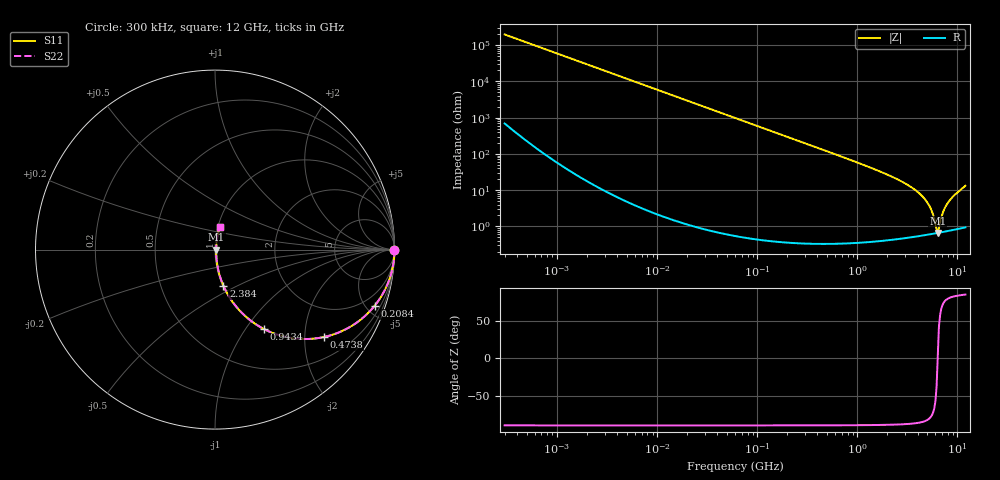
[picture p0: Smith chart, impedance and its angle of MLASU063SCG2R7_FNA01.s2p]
! MLASU063SCG2R7_FNA01  S-PARAMETER MODEL  ( Standard Model )
! Model Generated by TAIYO YUDEN Corporation (http://www.ty-top.com)
! Version 1.0
! TAIYO YUDEN Control No. 240819
! Copyright(c) 2024 TAIYO YUDEN CO.,LTD. All Rights Reserved.
! Product Description (link to TY-COMPAS)
! https://ds.yuden.co.jp/TYCOMPAS/or/detail?pn=MLASU063SCG2R7CFNA01&u=M
! Products Name : Multilayer Ceramic Capacitors
! Characteristics :
!  Capacitance : 2.7 [pF] , Rated Voltage : 50 [V] , TCC : CG / C0G
!  Case Size : 0.6 x 0.3 / 0.024 x 0.012 [mm/inch] , Thickness : 0.3 / 0.012 [mm/inch]
!  (Conditions: Temperature = 25 [degC] , DC Bias Voltage = 0 [V])
! External Node Assignments :
!  1  o---| |---o  2
! GND o---------o GND
! Frequency Range : 0.3MHz  -  12000MHz  [ 401 STEP ]
# MHZ S RI R 50
! Freq[MHz].  S11 Real  S11 Imag  S21 Real  S21 Imag  S12 Real  S12 Imag  S22 Real  S22 Imag
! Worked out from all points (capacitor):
!   401 points, 300 kHz to 12 GHz, reference 50 ohm
!   read as one part in series: C = 2.69 pF near 316.3 kHz
!   lowest |Z| = 658 mohm at 6.354 GHz (marker M1)
!   series resonance near 6.344 GHz, so ESL is about 230 pH
!   S11 on the Smith chart (normalised r, x): 300 kHz: open; 208.4 MHz: 1.01, -5.67; 473.8 MHz: 1.01, -2.48; 943.4 MHz: 1.01, -1.23; 2.384 GHz: 1.01, -0.43; 12 GHz: 1.02, +0.26
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0.3  1 -0.000508  2.04e-06 0.000508  2.04e-06 0.000508  1 -0.000508
1.769972  1 -0.00299  1.09e-05 0.00299  1.09e-05 0.00299  1 -0.00299
10.44266  0.9997 -0.0177  0.000319 0.0177  0.000319 0.0177  0.9997 -0.0177
60  0.9897 -0.1005  0.0103 0.1005  0.0103 0.1005  0.9897 -0.1005
208.3979  0.8889 -0.3137  0.1111 0.3137  0.1111 0.3137  0.8889 -0.3137
353.9943  0.7343 -0.4407  0.2657 0.4407  0.2657 0.4407  0.7343 -0.4407
473.7541  0.6059 -0.4874  0.3941 0.4874  0.3941 0.4874  0.6059 -0.4874
668.5285  0.4334 -0.4937  0.5666 0.4937  0.5666 0.4937  0.4334 -0.4937
943.3804  0.274 -0.4432  0.726 0.4432  0.726 0.4432  0.274 -0.4432
2088.533  0.0633 -0.2355  0.9367 0.2355  0.9367 0.2355  0.0633 -0.2355
2384.334  0.0472 -0.2021  0.9528 0.2021  0.9528 0.2021  0.0472 -0.2021
3547.679  0.0178 -0.1121  0.9822 0.1121  0.9822 0.1121  0.0178 -0.1121
4623.766  0.00916 -0.0593  0.9908 0.0593  0.9908 0.0593  0.00916 -0.0593
5278.635  0.00715 -0.0343  0.9928 0.0343  0.9928 0.0343  0.00715 -0.0343
5565.855  0.00672 -0.0245  0.9933 0.0245  0.9933 0.0245  0.00672 -0.0245
6026.253  0.00646 -0.0098  0.9935 0.0098  0.9935 0.0098  0.00646 -0.0098
6354.153  0.00653 0.000331  0.9935 -0.000331  0.9935 -0.000331  0.00653 0.000331
6699.894  0.00682 0.0106  0.9932 -0.0106  0.9932 -0.0106  0.00682 0.0106
7254.098  0.00763 0.0253  0.9924 -0.0253  0.9924 -0.0253  0.00763 0.0253
8064.993  0.00937 0.0443  0.9906 -0.0443  0.9906 -0.0443  0.00937 0.0443
9454.42  0.0135 0.073  0.9865 -0.073  0.9865 -0.073  0.0135 0.073
12000  0.0257 0.1267  0.9743 -0.1267  0.9743 -0.1267  0.0257 0.1267
